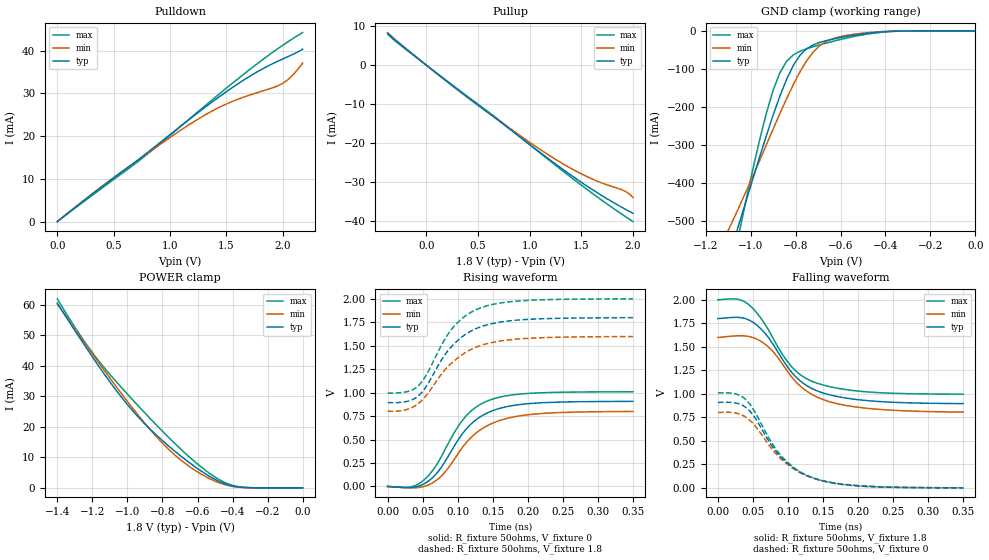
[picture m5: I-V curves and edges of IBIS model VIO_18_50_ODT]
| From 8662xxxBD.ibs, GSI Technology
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[Model]   VIO_18_50_ODT
Model_type   I/O
Polarity   Non-Inverting
Vinl  =   0.7000V
Vinh  =   1.1000V
Vmeas =   0.90v
Rref  =   50
|  variable   typ   min   max
C_comp   3.0pF   2.5pF   3.5pF
[Receiver Thresholds]
Vth = 0.90V
Vth_min = 0.80V
Vth_max = 0.95V
Threshold_sensitivity = 1.0
Reference_supply Ext_ref
Vinh_ac = +200mv
Vinh_dc = +100mv
Vinl_ac = -200mv
Vinl_dc = -100mv
Tslew_ac = 550ps
|  variable   typ   min   max
[External Reference]   0.90   0.80   0.95
|  variable   typ   min   max
[Temperature Range]   50   100   0
|  variable   typ   min   max
[Voltage Range]   1.8   1.6   2.0
[Add Submodel]
| Submodel Name   Mode
Strong_ODT_18V   Non-Driving
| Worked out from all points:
|   slope of the pulldown table from 0 to 0.27 V, typ, clamps not added: 48.3 ohm
|   slope of the pullup table from 0 to 0.27 V, typ, clamps not added: 48.1 ohm
|   GND clamp passes 1 mA (typ) near -0.36 V on its own axis
|   POWER clamp passes 1 mA (typ) near -0.43 V on its own axis
|   rising waveform, R_fixture 50ohms, V_fixture 0: 20-80 % time 54.4ps typ, 57.7ps min, 52.4ps max; typ from 0 V to 0.907 V
|   rising waveform, R_fixture 50ohms, V_fixture 1.8: 20-80 % time 54.6ps typ, 59.5ps min, 51.8ps max; typ from 0.894 V to 1.8 V
|   falling waveform, R_fixture 50ohms, V_fixture 1.8: 20-80 % time 59.2ps typ, 62.2ps min, 57ps max; typ from 1.8 V to 0.896 V
|   falling waveform, R_fixture 50ohms, V_fixture 0: 20-80 % time 59.3ps typ, 62.2ps min, 58.1ps max; typ from 0.908 V to 0.001 V
[Pullup]
| V(VDDQ-Vout)   typ   min   max
-376mV    8.242mA    8.399mA    8.053mA
-256mV    5.435mA    5.574mA    5.249mA
296mV     -6.144mA   -6.203mA   -5.985mA
680mV     -13.84mA   -13.76mA   -13.63mA
1.064V    -21.69mA   -20.98mA   -21.78mA
1.256V    -25.5mA    -24.28mA   -25.83mA
1.448V    -29.14mA   -27.2mA    -29.77mA
1.664V    -32.93mA   -29.9mA    -34.04mA
1.904V    -36.69mA   -32.14mA   -38.5mA
1.952V    -37.38mA   -32.83mA   -39.36mA
2V        -38.06mA   -34mA      -40.19mA
[PullDown]
| voltage   typ   min   max
0V        -7.795nA   -15.24nA   -7.985nA
374mV     7.698mA    7.792mA    7.395mA
726mV     14.64mA    14.52mA    14.24mA
1.166V    23.79mA    22.59mA    23.86mA
1.364V    27.77mA    25.71mA    28.24mA
1.518V    30.7mA     27.7mA     31.57mA
1.76V     34.79mA    30.03mA    36.62mA
1.98V     37.79mA    32.02mA    40.85mA
2.068V    38.83mA    33.67mA    42.4mA
2.112V    39.36mA    34.88mA    43.14mA
2.178V    40.32mA    37.09mA    44.21mA
[POWER Clamp]
|V(VDDQ-Vout)   typ   min   max
-1.4V     60.61mA    60.34mA    62.02mA
-1.288V   50.59mA    51.1mA     51.64mA
-1.204V   43.31mA    44.28mA    44.66mA
-1.008V   27.88mA    28.96mA    31.27mA
-924mV    22.38mA    22.81mA    26.03mA
-812mV    16.12mA    15.39mA    19.29mA
-672mV    9.383mA    8.076mA    11.45mA
-588mV    5.846mA    4.807mA    7.253mA
-504mV    2.89mA     2.285mA    3.677mA
-392mV    517.1uA    405.4uA    668.9uA
-308mV    61.99uA    56.59uA    69.17uA
0V        31.94nA    55.59nA    13.84nA
[GND Clamp]
|(Vout)   typ   min   max
-1.5V     -1.252A    -991.4mA   -1.695A
-1.11V    -618mA     -537.1mA   -698.9mA
-1.08V    -561.6mA   -499.5mA   -613.1mA
-1.05V    -504.3mA   -461mA     -527.9mA
-930mV    -275.4mA   -299.5mA   -216.8mA
-900mV    -221.7mA   -258.3mA   -156.7mA
-870mV    -171.8mA   -217.7mA   -110.4mA
-810mV    -90.76mA   -141.2mA   -63.07mA
-720mV    -36.41mA   -54.52mA   -41.49mA
-630mV    -21.21mA   -19.75mA   -26.99mA
-390mV    -1.828mA   -1.276mA   -2.431mA
0V        -7.821nA   -15.24nA   -8.228nA
[Ramp]
| voltage   typ   min   max
dV/dt_r   0.54/186p   0.48/213p   0.60/209p
dV/dt_f   0.86/129p   0.66/166p   1.07/101p
R_load  =   50ohms
[Rising Waveform]
R_fixture =   50ohms
V_fixture =   0
| Time   V(typ)   V(min)   V(max)
0s        190.1nV    366.4nV    199.4nV
35ps      -10.07mV   -14.67mV   -598.8uV
59.5ps    64.74mV    20.5mV     126.7mV
80.5ps    248.3mV    142.2mV    372mV
108.5ps   579.1mV    432.9mV    720.9mV
126ps     710.3mV    568.3mV    844.5mV
143.5ps   787.9mV    652.4mV    914.1mV
171.5ps   852.6mV    727.2mV    968.5mV
210ps     887.4mV    771.5mV    995.4mV
350ps     906.7mV    799.2mV    1.009V
[Rising Waveform]
R_fixture =   50ohms
V_fixture =   1.8
V_fixture_min =  1.6
V_fixture_max =  2.0
| Time   V(typ)   V(min)   V(max)
0s        894.4mV    802.3mV    996.1mV
24.5ps    901.9mV    813.9mV    1.006V
42ps      954mV      873.3mV    1.061V
52.5ps    1.037V     946mV      1.155V
77ps      1.35V      1.199V     1.508V
91ps      1.49V      1.313V     1.672V
112ps     1.625V     1.431V     1.823V
133ps     1.702V     1.503V     1.904V
196ps     1.778V     1.577V     1.981V
350ps     1.798V     1.597V     1.999V
[Falling Waveform]
R_fixture =   50ohms
V_fixture =   1.8
V_fixture_min = 1.6
V_fixture_max = 2.0
| Time   V(typ)   V(min)   V(max)
0s        1.8V       1.6V       2V
31.5ps    1.812V     1.618V     2.001V
52.5ps    1.749V     1.592V     1.888V
77ps      1.548V     1.463V     1.616V
105ps     1.232V     1.182V     1.29V
119ps     1.129V     1.073V     1.196V
136.5ps   1.048V     984.8mV    1.127V
164.5ps   981.1mV    906.1mV    1.069V
206.5ps   933.1mV    851.7mV    1.025V
350ps     896.3mV    806.1mV    996.9mV
[Falling Waveform]
R_fixture =   50ohms
V_fixture =   0
| Time   V(typ)   V(min)   V(max)
0s        908.3mV    801.5mV    1.01V
24.5ps    903.8mV    797mV      1.001V
38.5ps    863.9mV    758.2mV    948.5mV
52.5ps    750.7mV    665.5mV    811.7mV
73.5ps    487.6mV    448.7mV    520.6mV
87.5ps    347.3mV    326.5mV    365.4mV
108.5ps   208.4mV    199.7mV    215.3mV
133ps     113mV      110.8mV    113.7mV
199.5ps   22.8mV     25.01mV    20.12mV
350ps     639.9uV    1.036mV    374uV
